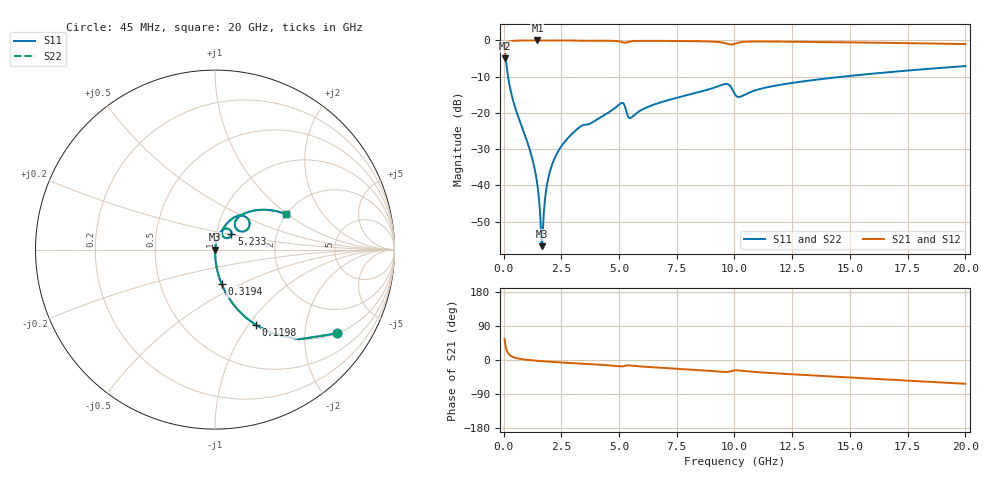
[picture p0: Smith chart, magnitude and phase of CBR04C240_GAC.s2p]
! S-parameter model data by Modelithics Inc.  support@modelithics.com 813-866-6335  Tampa FL USA
! S-Parameter data specifications:
! Substrate: 20-mil Rogers 4350B, substrate thickness, H=0.508mm, Dielectric constant, Er=3.75
! PCB Mounting Pad Footprint: Pad width, PadW=0.52mm , Pad length, PadL=0.52mm , Pad gap, PadG (edge-to-edge)=0.28mm , Reference planes=1.32mm apart
#  GHz  S  MA  R 50
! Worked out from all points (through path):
!   801 points, 45 MHz to 20 GHz, reference 50 ohm
!   highest |S21| = -0.01 dB at 1.467 GHz (marker M1); lowest = -5.0 dB at 45 MHz (marker M2)
!   group delay of S21, straight-line fit = 9.26 ps
!   lowest |S11| = -56.8 dB at 1.666 GHz (marker M3), VSWR 1.00, Z = 50.1 + j0.0226 ohm
!   |S11| at or under -10 dB: 195.1 MHz to 14.69 GHz (14.5 GHz wide, 195 % of centre)
!   |S22| runs from -56.8 to -1.7 dB; largest |S21 - S12| = 0
!   S11 on the Smith chart (normalised r, x): 45 MHz: 1.00, -2.92; 119.8 MHz: 1.00, -1.09; 319.4 MHz: 1.00, -0.40; 5.233 GHz: 1.18, +0.22; 20 GHz: 1.99, +0.98
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0.045  0.8257 -34.4  0.5638 55.6  0.5638 55.6  0.8257 -34.4
0.119831  0.4801 -61.5  0.8768 28.5  0.8768 28.5  0.4801 -61.5
0.194662  0.3168 -71.8  0.948 18.1  0.948 18.1  0.3168 -71.8
0.319381  0.195 -79.2  0.9802 10.7  0.9802 10.7  0.195 -79.2
1.192413  0.0269 -88.1  0.9984 -0.6  0.9984 -0.6  0.0269 -88.1
1.466794  0.01002 -84.5  0.9986 -2.1  0.9986 -2.1  0.01002 -84.5
1.591513  0.003654 -70.5  0.9986 -2.7  0.9986 -2.7  0.003654 -70.5
1.666344  0.001449 9.0  0.9985 -3.1  0.9985 -3.1  0.001449 9.0
1.741175  0.004098 65.9  0.9985 -3.4  0.9985 -3.4  0.004098 65.9
1.915781  0.01168 78.3  0.9983 -4.2  0.9983 -4.2  0.01168 78.3
2.165219  0.02184 80.4  0.998 -5.2  0.998 -5.2  0.02184 80.4
2.63915  0.03958 80.0  0.9971 -7.1  0.9971 -7.1  0.03958 80.0
3.387462  0.06657 73.9  0.9905 -10.0  0.9905 -10.0  0.06657 73.9
5.058694  0.1343 60.9  0.9625 -16.7  0.9625 -16.7  0.1343 60.9
5.2333  0.1282 44.3  0.93 -15.9  0.93 -15.9  0.1282 44.3
5.507681  0.08526 57.3  0.9702 -14.7  0.9702 -14.7  0.08526 57.3
6.704981  0.1366 67.8  0.9854 -20.0  0.9854 -20.0  0.1366 67.8
9.598456  0.2504 46.1  0.9161 -31.6  0.9161 -31.6  0.2504 46.1
10.0225  0.18 33.9  0.9004 -27.3  0.9004 -27.3  0.18 33.9
13.36496  0.2826 48.1  0.9531 -40.7  0.9531 -40.7  0.2826 48.1
16.68248  0.3646 37.4  0.9252 -51.7  0.9252 -51.7  0.3646 37.4
20  0.4425 26.5  0.8903 -62.8  0.8903 -62.8  0.4425 26.5
